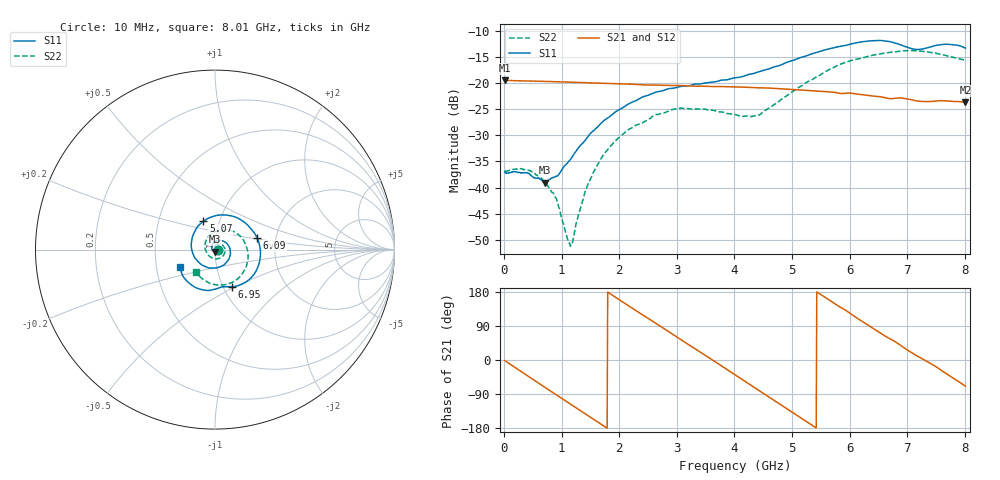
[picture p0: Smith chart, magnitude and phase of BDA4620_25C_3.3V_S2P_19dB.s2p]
!Agilent Technologies,E5071B,MY42404982,A.09.10
!Date: Wed May 06 08:52:47 2026
!Data & Calibration Information:
!Freq	S11:SOLT2(ON)	S21:SOLT2(ON)	S12:SOLT2(ON)	S22:SOLT2(ON)
# Hz S RI R 50
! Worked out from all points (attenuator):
!   801 points, 10 MHz to 8.01 GHz, reference 50 ohm
!   highest |S21| = -19.41 dB at 10 MHz (marker M1); lowest = -23.7 dB at 8.01 GHz (marker M2)
!   lowest |S11| = -39.0 dB at 710 MHz (marker M3), VSWR 1.02, Z = 49.8 - j1.09 ohm
!   |S11| at or under -10 dB: start of sweep to end of sweep
!   |S22| runs from -51.3 to -13.7 dB; largest |S21 - S12| = 0.00048
!   S11 on the Smith chart (normalised r, x): 10 MHz: 1.03, -0.00; 5.07 GHz: 0.84, +0.27; 6.09 GHz: 1.59, +0.22; 6.95 GHz: 1.10, -0.48; 8.01 GHz: 0.66, -0.14
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1e7  0.0141 -0.000922  0.107 -0.00232  0.1071 -0.00232  0.0143 -0.00053
4.3e8  0.00893 -0.0104  0.076 -0.0731  0.076 -0.0732  0.0136 -0.00551
7.1e8  -0.00202 -0.011  0.0321 -0.0994  0.0321 -0.0996  0.00832 -0.00767
9e8  -0.0103 -0.00753  -0.00216 -0.1037  -0.00229 -0.1039  0.00332 -0.00719
1.15e9  -0.0178 0.00499  -0.0455 -0.0921  -0.0456 -0.0923  -0.0023 -0.00148
1.19e9  -0.0185 0.0077  -0.0517 -0.0886  -0.0518 -0.0887  -0.003 -0.000159
1.35e9  -0.0187 0.0184  -0.0737 -0.0704  -0.0737 -0.0705  -0.00471 0.00515
1.56e9  -0.0123 0.0333  -0.0931 -0.0392  -0.0932 -0.0393  -0.00408 0.0137
1.82e9  0.00546 0.0469  -0.0998 0.00512  -0.0999 0.00519  0.00207 0.0238
2.15e9  0.039 0.0494  -0.08 0.0575  -0.0801 0.0576  0.018 0.0309
2.68e9  0.0832 0.00531  -0.00401 0.0961  -0.00389 0.0963  0.0467 0.0195
3.08e9  0.0767 -0.0534  0.0574 0.0761  0.0577 0.0761  0.0571 -0.00904
4.01e9  -0.0759 -0.0837  0.0719 -0.0583  0.0719 -0.0585  -0.013 -0.0485
4.42e9  -0.1292 -0.0031  0.0162 -0.0893  0.0161 -0.0895  -0.0481 -0.0127
5.07e9  -0.0652 0.1573  -0.0711 -0.0503  -0.0713 -0.0504  -0.0241 0.0847
5.35e9  0.0179 0.1919  -0.0842 -0.0111  -0.0842 -0.0112  0.0236 0.1062
6.09e9  0.2347 0.0646  -0.0328 0.0725  -0.033 0.0726  0.1633 0.0445
6.39e9  0.2497 -0.0596  0.0065 0.0754  0.00642 0.0755  0.1843 -0.0235
6.68e9  0.1873 -0.1699  0.0384 0.0605  0.0385 0.0606  0.1737 -0.0954
6.95e9  0.0944 -0.2067  0.061 0.0376  0.0611 0.0377  0.1352 -0.155
7.58e9  -0.0753 -0.2227  0.0613 -0.0299  0.0616 -0.0298  -0.0239 -0.1888
8.01e9  -0.1946 -0.0993  0.0235 -0.0612  0.0236 -0.0614  -0.1075 -0.1256
